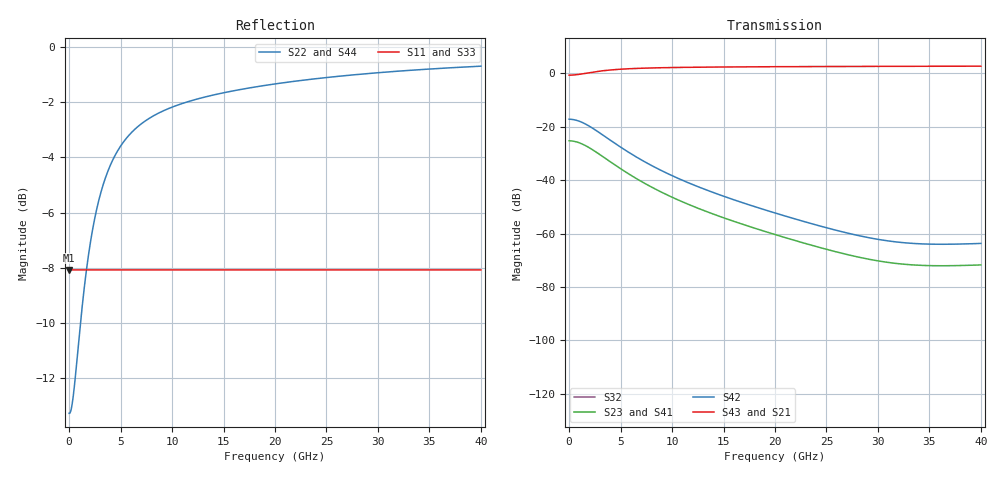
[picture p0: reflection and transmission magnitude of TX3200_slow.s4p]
# hz S ri R 50
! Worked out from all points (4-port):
!   20000 points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, 2 MHz to 40 GHz, reference 50 ohm
!   strongest paths, dB at 2 MHz, 10 GHz, 20 GHz, 30 GHz, 40 GHz:
!     S43: -0.7, 2.2, 2.5, 2.6, 2.7
!     S21: -0.8, 2.1, 2.4, 2.6, 2.7
!     S42: -17.2, -38.3, -52.3, -62.2, -63.7
!     S23: -25.3, -46.4, -60.4, -70.3, -71.8
!     S41: -25.3, -46.4, -60.4, -70.3, -71.8
!     S32: -, -, -, -, -
!   lowest |S11| = -8.1 dB at 2 MHz (marker M1), VSWR 2.30, Z = 115 + j0 ohm
!   |S11| at or under -10 dB: nowhere
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2000000  0.3945 0  0 0  0 0  0 0
         0.9144 0.000243  0.2169 -0.000616  -0.0545 7.06e-05  0.138 -0.000179
         0 0  0 0  0.3945 0  0 0
         -0.0545 7.06e-05  0.138 -0.000179  0.9211 0.000235  0.2 -0.000597
1.464e9  0.3945 0  0 0  0 0  0 0
         0.9755 0.1418  0.062 -0.3595  -0.0295 0.0346  0.0748 -0.0878
         0 0  0 0  0.3945 0  0 0
         -0.0295 0.0346  0.0748 -0.0878  0.9791 0.1387  0.053 -0.3515
2.842e9  0.3945 0  0 0  0 0  0 0
         1.07 0.1941  -0.1785 -0.492  -0.00257 0.0313  0.00651 -0.0793
         0 0  0 0  0.3945 0  0 0
         -0.00257 0.0313  0.00652 -0.0793  1.071 0.1926  -0.1809 -0.4883
5.574e9  0.3945 0  0 0  0 0  0 0
         1.192 0.1894  -0.4865 -0.4802  0.00848 0.011  -0.0215 -0.0278
         0 0  0 0  0.3945 0  0 0
         0.00848 0.011  -0.0215 -0.0278  1.194 0.191  -0.4921 -0.4842
9.438e9  0.3945 0  0 0  0 0  0 0
         1.262 0.1544  -0.6634 -0.3914  0.00493 0.00214  -0.0125 -0.00542
         0 0  0 0  0.3945 0  0 0
         0.00493 0.00214  -0.0125 -0.00543  1.266 0.155  -0.6754 -0.3928
2.7748e10  0.3945 0  0 0  0 0  0 0
           1.339 0.0907  -0.8604 -0.2299  0.000227 -0.000297  -0.000576 0.000754
           0 0  0 0  0.3945 0  0 0
           0.000228 -0.000296  -0.000578 0.00075  1.341 0.0877  -0.8639 -0.2222
4e10  0.3945 0  0 0  0 0  0 0
      1.357 0.0731  -0.9042 -0.1854  -0.000154 -0.000207  0.000389 0.000526
      0 0  0 0  0.3945 0  0 0
      -0.000153 -0.000207  0.000387 0.000525  1.357 0.0712  -0.9044 -0.1805
